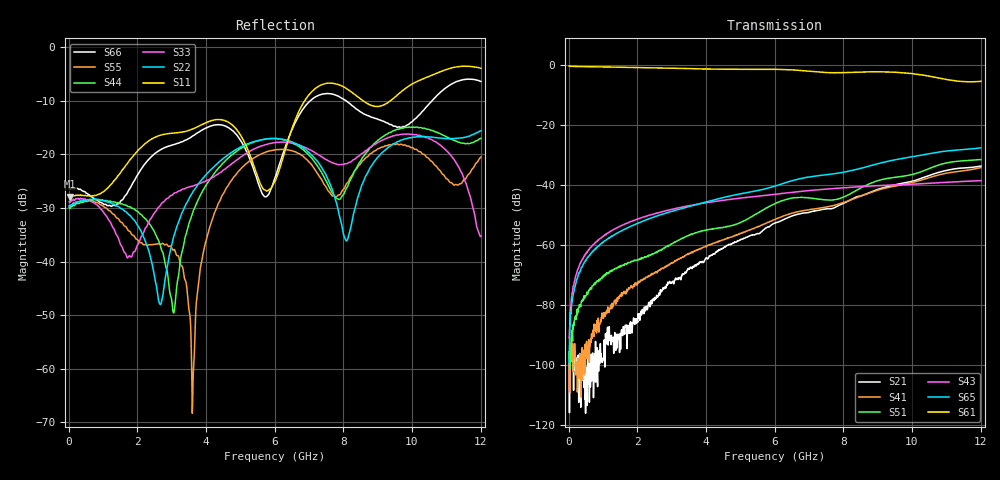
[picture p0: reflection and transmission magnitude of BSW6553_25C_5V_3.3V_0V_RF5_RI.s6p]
! Agilent Technologies	N5230C	MY49001333	A.09.33.09
!	Test time	=	2026-05-26
!	Product	=	BSW6553
!	Temp	=	25C
!	Logic	=	RF5
!	Port1	=	RFC
!	Port2	=	RF1
!	Port3	=	RF2
!	Port4	=	RF3
!	Port5	=	RF4
!	Port6	=	RF5
!S6P File: Measurements: <S11,S12,S13,S14,S15,S16>,
!<S21,S22,S23,S24,S25,S26>,
!<S31,S32,S33,S34,S35,S36>,
!<S41,S42,S43,S44,S45,S46>,
!<S51,S52,S53,S54,S55,S56>,
!<S61,S62,S63,S64,S65,S66>;
# HZ S RI R 50
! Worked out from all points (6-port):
!   1201 points, 10 MHz to 12.01 GHz, reference 50 ohm
!   strongest paths, dB at 10 MHz, 3.01 GHz, 6.01 GHz, 9.01 GHz, 12.01 GHz:
!     S61: -0.5, -1.2, -1.6, -2.4, -5.6
!     S65: -99.0, -48.8, -40.4, -32.9, -27.7
!     S43: -90.8, -48.1, -43.1, -40.3, -38.6
!     S51: -95.4, -59.6, -46.2, -38.6, -31.6
!     S41: -99.6, -65.9, -51.5, -41.7, -34.2
!     S21: -96.3, -72.5, -52.7, -41.5, -33.7
!   lowest |S11| = -27.9 dB at 40 MHz (marker M1), VSWR 1.08, Z = 54.2 - j0.477 ohm
!   |S11| at or under -10 dB: start of sweep to 6.873 GHz; 8.581 GHz to 9.369 GHz (787.1 MHz wide, 8.77 % of centre)
